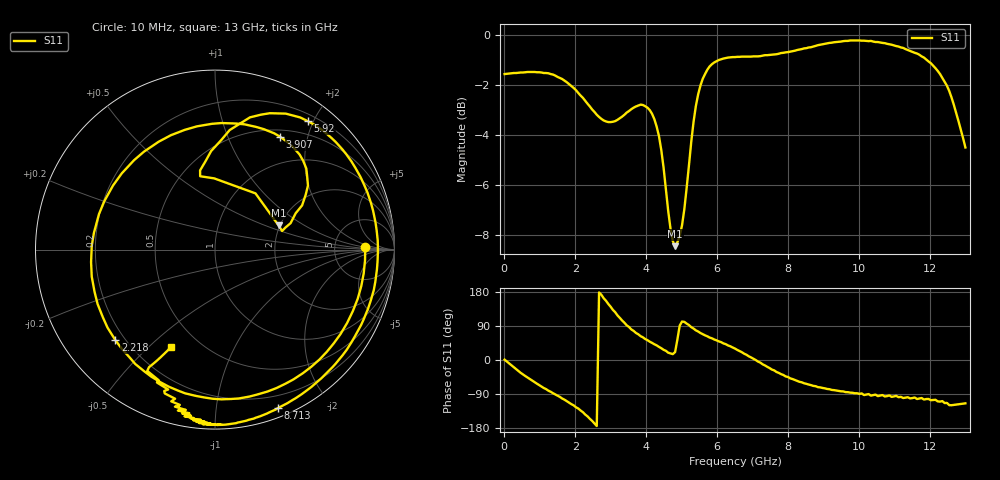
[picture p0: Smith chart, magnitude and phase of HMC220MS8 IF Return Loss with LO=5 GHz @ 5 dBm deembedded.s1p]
!Hittite Microwave Corporation
!12 Elizabeth Drive
!Chelmsford, MA 01824
!Tel: 978-250-3343
!Fax: 978-250-3373
!Device: HMC220MS8, 5-12 GHz, GaAS MMIC SMT Double-Balanced Mixer in 8-lead MSOP package
!Misc: IF Return Loss, LO = 5 GHz @ 5dBm, Room
# MHZ S MA R 50
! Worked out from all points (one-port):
!   201 points, 10 MHz to 13 GHz, reference 50 ohm
!   lowest |S11| = -8.4 dB at 4.816 GHz (marker M1), VSWR 2.22, Z = 98.4 + j31 ohm
!   |S11| at or under -10 dB: nowhere
!   S11 on the Smith chart (normalised r, x): 10 MHz: 11, +1; 2.218 GHz: 0.16, -0.38; 3.907 GHz: 0.59, +1.57; 5.92 GHz: 0.30, +1.92; 8.713 GHz: 0.08, -1.47; 13 GHz: 0.35, -0.59
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10  0.837 0.9
464.65  0.843 -34.0
854.35  0.845 -58.9
1244.05  0.84 -80.9
1633.75  0.818 -101.7
2218.3  0.75 -137.7
2737.9  0.681 172.1
3257.5  0.683 111.1
3517.3  0.706 87.1
3907  0.726 60.0
4361.65  0.629 34.6
4621.45  0.446 19.3
4816.3  0.379 20.9
4881.25  0.386 54.2
4946.2  0.397 90.7
5076.1  0.449 100.7
5465.8  0.762 75.2
5920.45  0.883 54.1
6505  0.905 30.2
7219.45  0.909 -7.0
7674.1  0.917 -31.6
8128.75  0.93 -50.3
8713.3  0.95 -68.4
9752.5  0.977 -86.1
11376.25  0.935 -98.2
12350.5  0.822 -108.5
12545.35  0.774 -119.2
13000  0.597 -114.4
